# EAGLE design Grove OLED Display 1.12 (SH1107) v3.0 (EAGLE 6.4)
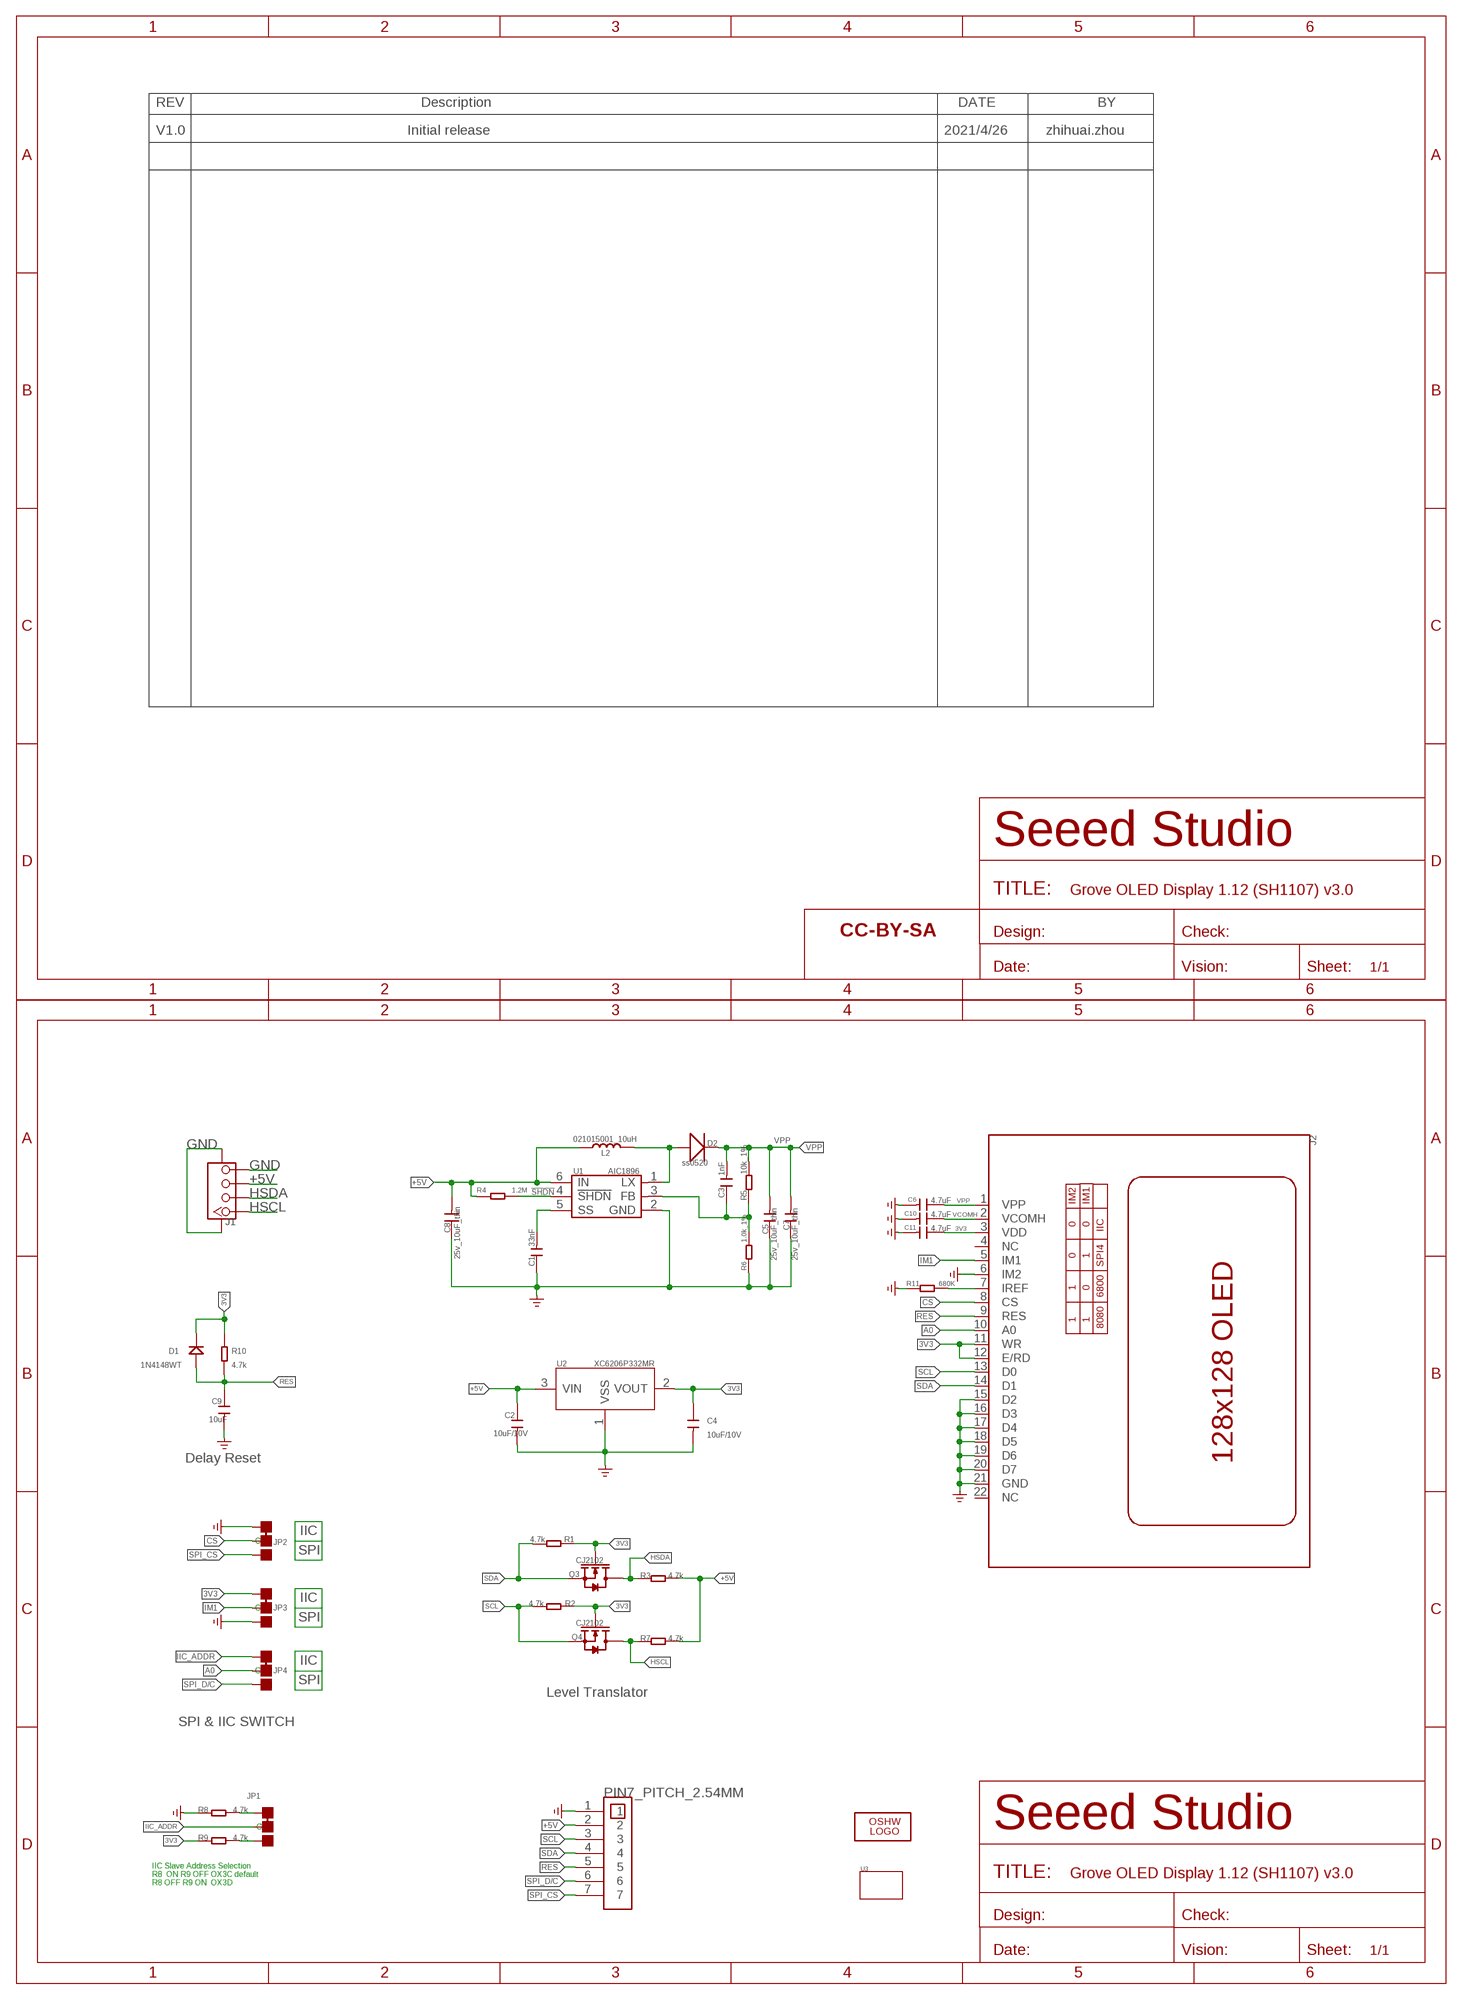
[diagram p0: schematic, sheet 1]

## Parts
C1  33nF  C-0603  [C0603]
C2  10uF/10V  C-0603  [C0603]
C3  1nF  C-0603  [C0603]
C4  10uF/10V  C-0603  [C0603]
C5  25v_10uF_thin  CAP-0805  [C0805]
C6  4.7uF  CAP-0603  [C0603]
C7  25v_10uF_thin  CAP-0805  [C0805]
C8  25v_10uF_thin  006-C0805  [0805]
C9  10uF  C-0603  [C0603]
C10  4.7uF  CAP-0603  [C0603]
C11  4.7uF  CAP-0603  [C0603]
D1  1N4148WT  DIODE'0603'  [SOD-523]
D2  ss0520  010-DSOD123  [SOD123]
FR1  SEEEDSTUDIO-OPEN-SCH-FRAME  [SEEEDSTUDIO-PCB-FRAME]
J1  TWIG-4P-2.0-SMD-FEMALE-REINFORCE'90D'  [4P-SMD-2.0-90D]
J2  OLED-128128-22P  [OLED22P-0.7]
JP1  JP-3P-SHORT  [3P-SMD-SHORT]
JP2  JP-3P-SHORT  [3P-SMD-SHORT]
JP3  JP-3P-SHORT  [3P-SMD-SHORT]
JP4  JP-3P-SHORT  [3P-SMD-SHORT]
L2  021015001_10uH  013-L0806  [0806]
LOGO2  LOGO-OSHW-FILLX0200-NT  [OSHW_FILLX200_NOTEXT]
Q3  CJ2102  MOSFET-N'SI1304BDL'  [SOT-323]
Q4  CJ2102  MOSFET-N'SI1304BDL'  [SOT-323]
R1  4.7k  R-0603  [R0603]
R2  4.7k  R-0603  [R0603]
R3  4.7k  R-0603  [R0603]
R4  1.2M  R-0603  [R0603]
R5  10k_1%  R-0603  [R0603]
R6  1.0k_1%  R-0603  [R0603]
R7  4.7k  R-0603  [R0603]
R8  4.7k  R-0603  [R0603]
R9  4.7k  R-0603  [R0603]
R10  4.7k  R-0603  [R0603]
R11  680K  R-0603  [R0603]
U1  AIC1896  [SOT23-6]
U2  XC6206P332MR  PMIC-XC6206PMR  [SOT-23]
U3  GROVE_OLED  [GROVE_OLED]
U$4  PIN7_PITCH_2.54MM  [PIN7_PITCH_2.54MM]

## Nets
3V3: C4.1 C11.1 D1.- J2.3(VDD) J2.11(WR) J2.12(E/RD) JP3.11(L) Q3.1(G) Q4.1(G) R1.1 R2.2 R9.1 R10.2 U2.2(VOUT)
!SHDN: R4.2 U1.4(!SHDN)
+5V: C2.1 C8.2 J1.3 L2.1 R3.2 R4.1 R7.2 U1.6(IN) U2.3(VIN) U$4.2
A0: J2.10(A0) JP4.MM(C)
CS: J2.8(CS) JP2.MM(C)
GND: C1.1 C2.2 C4.2 C5.1 C6.2 C7.1 C8.1 C9.2 C10.2 C11.2 J1.4 J1.SS1 J1.SS2 J2.6(IM2) J2.15(D2) J2.16(D3) J2.17(D4) J2.18(D5) J2.19(D6) J2.20(D7) J2.21(GND) JP2.11(L) JP3.00(R) R6.1 R8.1 R11.1 U1.2(GND) U2.1(VSS) U$4.1 ; supply symbol labelled GND_POWER
HSCL: J1.1 Q4.3(D) R7.1
HSDA: J1.2 Q3.3(D) R3.1
IIC_ADDR: JP1.MM(C) JP4.11(L)
IM1: J2.5(IM1) JP3.MM(C)
N$1: D2.+ L2.2 U1.1(LX)
N$2: C1.2 U1.5(SS)
N$3: J2.7(IREF) R11.2
N$4: C3.1 R5.1 R6.2 U1.3(FB)
N$10: JP1.11(L) R8.2
N$11: JP1.00(R) R9.2
RES: C9.1 D1.+ J2.9(RES) R10.1 U$4.5
SCL: J2.13(D0) Q4.2(S) R2.1 U$4.3
SDA: J2.14(D1) Q3.2(S) R1.2 U$4.4
SPI_CS: JP2.00(R) U$4.7
SPI_D/C: JP4.00(R) U$4.6
VCOMH: C10.1 J2.2(VCOMH)
VPP: C3.2 C5.2 C6.1 C7.2 D2.- J2.1(VPP) R5.2
Unconnected: J2.4(NC) J2.22(NC)

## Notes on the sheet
- V1.0 | Initial release | 2021/4/26 | zhihuai.zhou
- Delay Reset
- IIC
- SPI
- IIC
- SPI
- IIC
- SPI
- Level Translator
- SPI & IIC SWITCH
- IIC Slave Address Selection
- R8  ON R9 OFF OX3C default
- R8 OFF R9 ON  OX3D

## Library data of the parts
C1-C4 C9 = Discrete-small:C*: Ceramic Capacitors
C5-C7 C10 C11 = Discrete-new:CAP: Ceramic Capacitors
C8 = Discrete:006-C*: Ceramic Capacitors
D1 = Discrete-new:DIODE
D2 = Discrete:010-D*
FR1 = moudle-new:SEEEDSTUDIO-OPEN-SCH-FRAME
J1 = Connector:TWIG-4P-2.0-SMD-FEMALE-REINFORCE
J2 = OLED-128x128-22P:OLED-128*128-22P: ZJY-2828TSWIG01
JP1-JP4 = Discrete-new:JP-3P-SHORT
L2 = Discrete:013-L*
LOGO2 = logo:LOGO-OSHW-FILL; PARTNO: DNP
Q3 Q4 = Discrete-new:MOSFET-N: IRLL014: http://www.vishay.com/docs/91319/sihll014.pdf
R1-R11 = Discrete-small:R*
U1 = ICs_v54:AIC1896
U2 = IC-new:PMIC-XC6206P: LOW ESR Cap.Compatible Positive Voltage Regulators
U3 = Grove_oled:GROVE_OLED
U$4 = PIN_PITCH_2.54MM:PIN7_PITCH_2.54MM

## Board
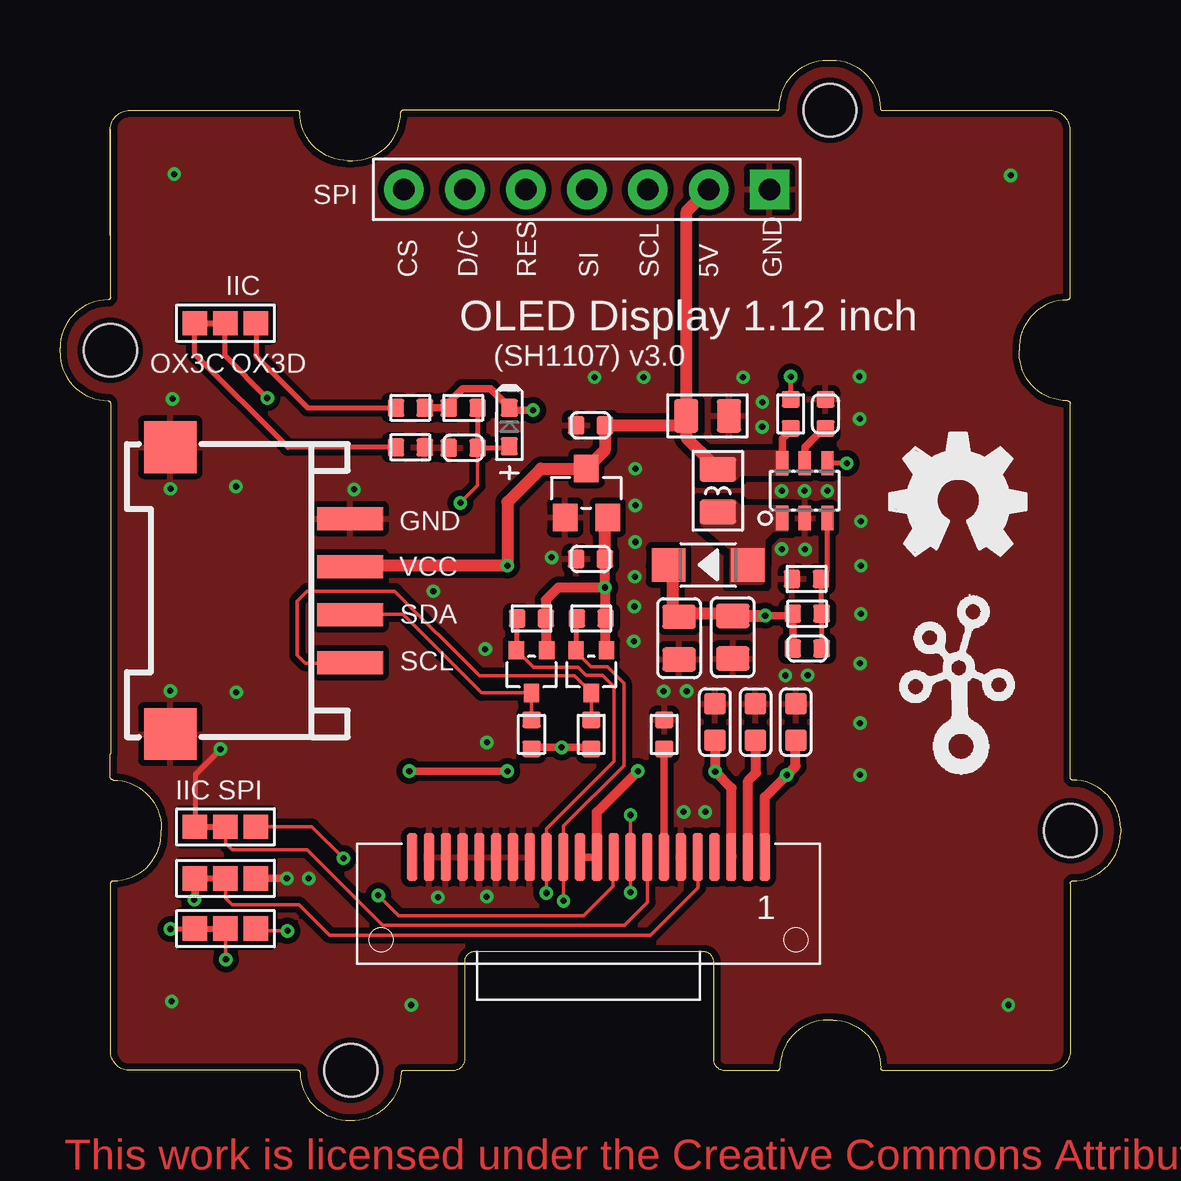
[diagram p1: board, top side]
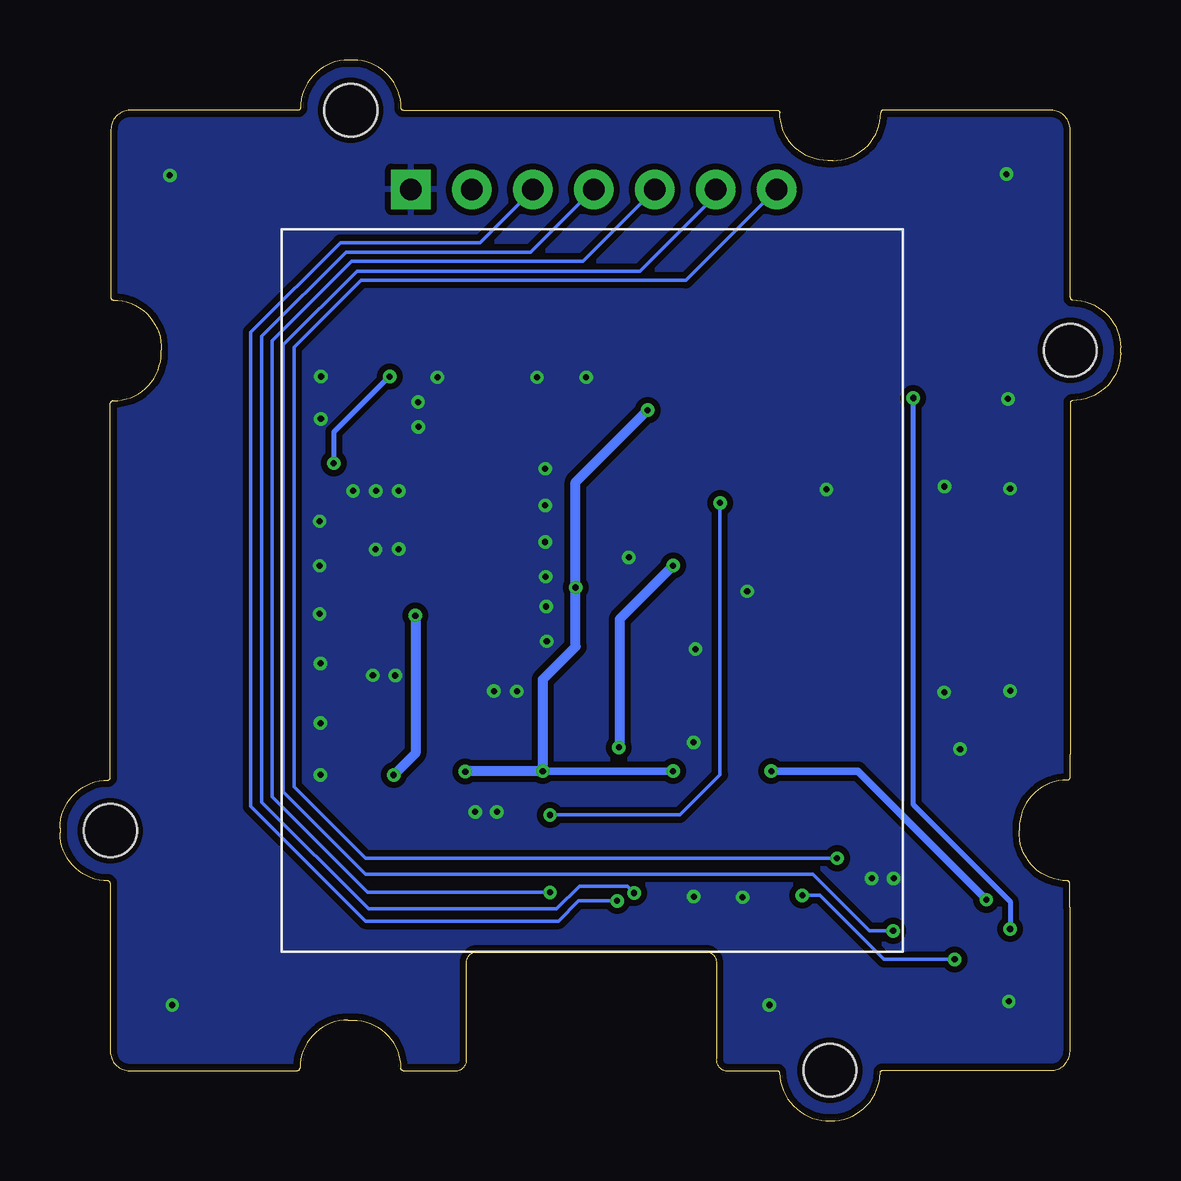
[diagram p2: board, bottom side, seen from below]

Size 44.21 x 44.2 mm. Coordinates in mm from the lower left corner, seen from the top.
Copper layers (1*16): Top 0.035mm / dielectric 1.5mm / Bottom 0.035mm
Design rules "SeeedStudio_2layer_DRU_no_angle_20140221 *": minimum track width 6mil, minimum drill 10mil, track to track 6mil, track to pad 6mil, pad to pad 6mil, via to via 6mil, smd to smd 0mil, copper to edge 10mil, drill to drill 10mil, minimum pad ring 10mil, minimum via ring 6mil, stop-mask expansion 2mil, vias tented up to drill 25mil, thermal gap 10mil

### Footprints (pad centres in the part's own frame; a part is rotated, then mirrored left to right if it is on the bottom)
C0603 = smd 0.696 x 0.762: 1 0.602,0; 2 -0.602,0
C0805 = smd 1.397 x 1.016: 1 0,0.889; 2 0,-0.889
C0603' = smd 0.889 x 0.889: 1 0,0.762; 2 0,-0.762
0805 = smd 1.016 x 1.397: 1 -0.889,0; 2 0.889,0
SOD-523 = smd 0.762 x 0.7: + 0.8,0; - -0.8,0
SOD123 = smd 1.397 x 1.397: + 1.651,0; - -1.651,0
4P-SMD-2.0-90D = smd 0.965 x 2.74: 1 -3,-0.1; 2 -1,-0.1; 3 1,-0.1; 4 3,-0.1 | smd 2.159 x 2.184: SS1 -5.974,7.4; SS2 5.974,7.4
OLED22P-0.7 = smd 0.4 x 2 bottom: 1 -7.35,-11.1; 2 -6.65,-11.1; 3 -5.95,-11.1; 4 -5.25,-11.1; 5 -4.55,-11.1; 6 -3.85,-11.1; 7 -3.15,-11.1; 8 -2.45,-11.1; 9 -1.75,-11.1; 10 -1.05,-11.1; 11 -0.35,-11.1; 12 0.35,-11.1; 13 1.05,-11.1; 14 1.75,-11.1; 15 2.45,-11.1; 16 3.15,-11.1; 17 3.85,-11.1; 18 4.55,-11.1; 19 5.25,-11.1; 20 5.95,-11.1; 21 6.65,-11.1; 22 7.35,-11.1
3P-SMD-SHORT = smd 1.016 x 1.016: 00 -1.27,0; 11 1.27,0; MM 0,0
0806 = smd 1.016 x 1.524: 1 -0.889,0; 2 0.889,0
SOT-323 = smd 0.762 x 0.635: 1 0.889,-0.635; 2 0.889,0.635; 3 -0.889,0
R0603 = smd 0.696 x 0.762: 1 0.602,0; 2 -0.602,0
SOT23-6 = smd 0.508 x 1.016: 1 -0.94,-1.143; 2 0,-1.143; 3 0.94,-1.143; 4 0.94,1.143; 5 0,1.143; 6 -0.94,1.143
SOT-23 = smd 1.016 x 1.143: 1 -0.889,-1.016; 2 0.889,-1.016; 3 0,1.016
GROVE_OLED = hole 2.2: -19.955,10.015; 10.033,20.01; 20.055,-9.995; -9.933,-19.99
PIN7_PITCH_2.54MM = drill 0.889 pad 1.651 square: 1 0,0 | drill 0.889 pad 1.651: 2 0,-2.54; 3 0,-5.08; 4 0,-7.62; 5 0,-10.16; 6 0,-12.7; 7 0,-15.24

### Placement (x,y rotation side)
C1  31.91,29.46 90 top
C2  22.12,28.98 0 top
C3  31.15,19.68 0 top
C4  22.12,23.41 0 top
C5  28.04,20.15 180 top
C6  4.7uF  [C0603']  30.67,16.61 180 top
C7  25.81,20.11 180 top
C8  26.99,29.37 180 top
C9  16.81,28.04 0 top
C10  4.7uF  [C0603']  29,16.61 180 top
C11  4.7uF  [C0603']  27.3,16.61 180 top
D1  18.73,28.91 270 top
D2  27.02,23.16 0 top
FR1  not placed on the board
J1  12,22.09 90 top
J2  22.03,22.09 0 bottom
JP1  6.9,33.23 180 top
JP2  6.9,12.25 180 top
JP3  6.9,10.1 180 top
JP4  6.9,8.01 180 top
L2  27.42,26.25 270 top
LOGO2  34.6,23.56 0 top
Q3  19.66,18.72 90 top
Q4  22.15,18.72 90 top
R1  19.66,20.93 0 top
R2  22.15,20.93 180 top
R3  19.66,16.1 90 top
R4  30.46,29.46 270 top
R5  31.15,21.13 0 top
R6  31.12,22.58 180 top
R7  22.15,16.1 90 top
R8  14.61,28.06 0 top
R9  14.61,29.71 0 top
R10  16.81,29.71 0 top
R11  25.19,16.1 90 top
U1  31.04,26.25 0 top
U2  21.94,26.16 0 top
U3  22.05,22.09 0 top
U$1  [TWIGLOGO]  37.5,15.4 0 top
U$4  29.58,38.81 270 top

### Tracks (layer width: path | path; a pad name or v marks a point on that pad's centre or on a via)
3V3  (via drill 0.25 pad 0.51)
  Top 0.305: 28,11.01 J2.3 | R9.1 R10.2 16.24,29.74 16.24,29.96 16.77,30.5 17.94,30.5 D1.- | J2.12 J2.11 | D1.- | D1.- 18.73,29.64 | v19.72,29.61 18.83,29.61 D1.- | v18.65,14.57 v14.56,14.57 | v5.6,9.21 5.63,9.21 JP3.11
  Top 0.406: Q4.1 22.75,19.64 R2.2 | Q3.1 20.26,19.64 R1.1 20.25,21.71 20.76,22.22 v22.72,22.22 | 28,11.01 28,13.86 v27.31,14.55 27.31,15.84 C11.1 | J2.11 22.38,12.86 v24.09,14.57 | 22.71,20.96 R2.2 | R2.2 22.72,20.96 v22.72,22.22 C4.1
  Top 0.508: C4.1 22.72,25.03 U2.2
  Bottom 0.305: v18.65,14.57 v24.09,14.57 | v14.56,14.57 10.96,14.57 v5.6,9.21
  Bottom 0.406: v27.31,14.55 27.29,14.57 v24.09,14.57 24.09,18.38 22.72,19.75 v22.72,22.22 22.72,26.61 v19.72,29.61
!SHDN  (via drill 0.25 pad 0.51)
  Top 0.203: R4.2 v30.46,31 | v32.8,27.4 U1.4
  Bottom 0.203: v30.46,31 30.49,31 32.8,28.69 v32.8,27.4
+5V  (via drill 0.25 pad 0.51)
  Top 0.305: R3.2 19.72,15.56 v20.91,15.56 22.08,15.56 R7.2 | 30.16,27.7 30.21,27.65 30.21,27.4 30.18,27.4 30.16,27.37 30.13,27.4 U1.6 30.11,28.41 30.36,28.67 30.36,28.88 R4.1
  Top 0.508: J1.3 | L2.1 27.19,27.37 26.12,28.44 26.12,29.36 | 26.12,29.36 C8.2 | 26.12,29.36 26.12,37.89 U$4.2 | C8.2 26.11,28.96 26.09,28.95 | C8.2 25.71,28.98 C2.1 22.72,27.95 U2.3 20.05,27.17 18.65,25.77 v18.65,23.13 12.14,23.13 J1.3 | 12.11,23.11 J1.3
  Bottom 0.406: v20.91,15.56 20.89,15.59 20.89,20.9 v18.65,23.13
  pour Top (isolate 0.254, no thermals): 30.34,27.91 27.02,27.91 26.68,27.58 26.68,26.71 26.76,26.64 28.13,26.64 28.39,26.89 30.32,26.89 30.34,26.92
A0  (via drill 0.25 pad 0.51)
  Top 0.152: v13.27,9.39 14.1,8.55 21.83,8.55 23.05,9.77 23.05,10.96 J2.10 | v6.92,6.72 6.92,7.86 JP4.MM
  Bottom 0.152: v13.27,9.39 12.53,9.39 9.86,6.72 v6.92,6.72
CS
  Top 0.152: JP2.MM 6.9,11.57 7.17,11.29 10.29,11.29 13.44,8.14 23.53,8.14 24.49,9.11 24.49,10.98 J2.8 24.44,10.95
GND  (via drill 0.25 pad 0.51)
  Top 0.152: 6.9,12.25 5.71,12.25 5.65,12.18
  Top 0.203: 5.65,12.18 5.65,14.44 v6.69,15.49
  Top 0.305: JP3.00 v9.46,10.1 | v9.46,10.1
  other vias: 23.99,24.12 33.39,21.12 31.04,26.25 28.48,30.98 4.61,26.33 7.34,26.43 31.05,23.81 22.28,30.98 4.69,30.08 29.27,28.91 33.35,14.41 33.35,16.57 33.35,19.06 7.35,17.86 30.24,18.55 33.33,31.01 31.17,18.57 25.99,12.87 4.6,17.91 33.39,24.98 33.39,23.13 29.28,29.94 20.5,23.47 33.34,29.25 12.26,26.31 24.33,30.98 25.16,17.9 30.09,26.25 23.94,21.43 26.12,17.9 30.09,23.82 26.9,12.87 23.96,22.67 17.8,15.77 23.92,19.98 23.99,25.65 31.99,26.25 23.99,27.17 10.37,10.1 15.76,9.31 17.79,9.34 17.72,19.65 15.56,22.06 14.64,4.83 4.66,4.98 39.53,4.83 39.63,39.4 4.76,39.45
  pour Top (isolate 0.254, rank 2): -0.2,-0.14 44.25,0.25 44.25,44.7 -0.2,44.31
  pour Bottom (isolate 0.254, rank 6): -0.2,-0.14 44.25,-0.14 44.25,44.31 -0.2,44.31
HSCL
  Top 0.152: 11.69,19.09 11.51,18.91 11.92,18.91 J1.1 | J1.1 | J1.1 12.07,19.07 10.22,19.07 9.89,19.4 9.89,21.66 10.29,22.07 13.95,22.07 17.48,18.53 21.45,18.53 Q4.3 R7.1
  Top 0.406: 12.14,19.04 J1.1
HSDA
  Top 0.152: J1.2 14.31,21.1 17.58,17.83 Q3.3 R3.1
IIC_ADDR  (via drill 0.25 pad 0.51)
  Top 0.203: v8.64,30.12 6.89,31.87 JP1.MM | v4.61,7.99 5.6,7.99 JP4.11
  Bottom 0.203: v8.64,30.12 8.64,13.18 4.61,9.14 v4.61,7.99
IM1
  Top 0.152: J2.5 26.6,10.97 26.6,9.72 24.62,7.74 11.23,7.74 9.96,9.01 7.17,9.01 6.92,9.26 6.92,10.08 JP3.MM
N$1
  pour Top (isolate 0.254, no thermals): 30.37,25.62 28.39,25.62 28.13,25.88 26.79,25.88 26.68,25.78 26.68,24.89 27.93,23.79 27.9,22.42 27.98,22.35 29.28,22.35 29.38,22.47 29.4,24.23 29.73,24.56 30.32,24.56 30.37,24.61
N$2
  Top 0.305: C1.2 31.84,28.85 31.05,28.06 U1.5
N$3
  Top 0.305: J2.7 R11.2
N$4
  Top 0.203: 31.89,25.02 U1.3 31.99,22.9 31.72,22.67 R6.2 31.75,22.55 R5.1 C3.1
N$10
  Top 0.203: R8.2 9.51,28.06 5.62,31.95 JP1.11 | 6.89,33.22 6.9,33.23
N$11
  Top 0.152: 8.19,33.25 JP1.00
  Top 0.203: JP1.00 8.17,31.86 10.32,29.71 R9.2
RES  (via drill 0.25 pad 0.51)
  Top 0.152: v23.78,9.52 23.81,10.96 J2.9 v23.78,12.74 | 17.43,28.02 C9.1 17.41,26.48 16.7,25.77 v16.7,25.75
  Top 0.203: R10.1 C9.1 18.66,28.04 D1.+
  Bottom 0.152: v23.78,12.74 18.37,12.74 16.7,14.42 v16.7,25.75 | v23.78,9.52 31.38,9.52 35.36,13.5 35.36,32.5 32.06,35.81 22.41,35.81 19.42,38.8 U$4.5
SCL  (via drill 0.25 pad 0.51)
  Top 0.152: Q4.2 21.51,19.54 22.13,18.91 22.82,18.91 23.5,18.23 23.5,14.8 20.99,12.29 20.99,11.52 21.01,11.5 21.01,11.02 J2.13 v20.99,9.16
  Top 0.203: R2.1 21.51,20.67 Q4.2
  Bottom 0.152: v20.99,9.16 22.59,9.16 23.43,8.32 31.48,8.32 36.25,13.1 36.25,32.86 32.52,36.59 26.7,36.59 24.5,38.8 U$4.3
SDA  (via drill 0.25 pad 0.51)
  Top 0.152: 19.02,19.56 Q3.2 19.74,18.89 21.6,18.89 21.93,18.56 22.61,18.56 23.1,18.08 23.1,14.98 20.28,12.16 J2.14 v20.28,9.49
  Top 0.203: R1.2 19.02,20.67 Q3.2
  Bottom 0.152: v20.28,9.49 20.56,9.77 22.56,9.77 23.5,8.83 31.35,8.83 35.8,13.28 35.8,32.68 32.29,36.19 24.59,36.19 21.97,38.81 U$4.4
SPI_CS  (via drill 0.25 pad 0.51)
  Top 0.152: v11.82,10.94 10.5,12.26 JP2.00
  Top 0.203: JP2.00 8.25,12.25 8.31,12.18
  Bottom 0.152: v11.82,10.94 31.48,10.94 34.45,13.91 34.45,32.23 31.66,35.02 18.12,35.02 14.34,38.8 U$4.7
SPI_D/C  (via drill 0.25 pad 0.51)
  Top 0.152: v9.48,7.92 8.21,7.92
  Top 0.305: 8.21,7.92 JP4.00
  Bottom 0.152: U$4.6 16.88,38.54 20.02,35.4 31.83,35.4 34.91,32.33 34.91,13.71 31.48,10.28 12.83,10.28 10.47,7.92 v9.48,7.92
VCOMH
  Top 0.406: J2.2 28.68,14.16 29.01,14.5 29.01,15.83 C10.1
VPP  (via drill 0.25 pad 0.51)
  Top 0.305: C3.2 R5.2 30.45,21.04 29.38,21.04
  Top 0.406: J2.1 29.38,13.49 v30.3,14.41 30.67,14.77 C6.1
  Top 0.508: C5.2 28.04,21.13 25.81,21.13 C7.2 | 24.93,23.13 D2.- 25.51,23.16 25.53,23.13 25.53,21.27 C7.2 | 28.14,21.13 C5.2 | C5.2 29.38,21.04 v29.4,21.05 | C7.2 25.51,21 25.46,21.05
  Bottom 0.406: v29.4,21.05 29.4,15.31 v30.3,14.41

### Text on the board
tPlace: OLED Display 1.12 inch | (SH1107) v3.0
tNames: SPI | CS | D/C | RES | SI | SCL | 5V | GND | IIC | OX3C | OX3D | GND | VCC | SDA | SCL | IIC SPI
